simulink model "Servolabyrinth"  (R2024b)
settings: Solver=FixedStepAuto  StartTime=0.0  StopTime=inf  FixedStep=0.01  RelTol=1e-3  EnableMultiTasking=on
libraries: arduinolib x8

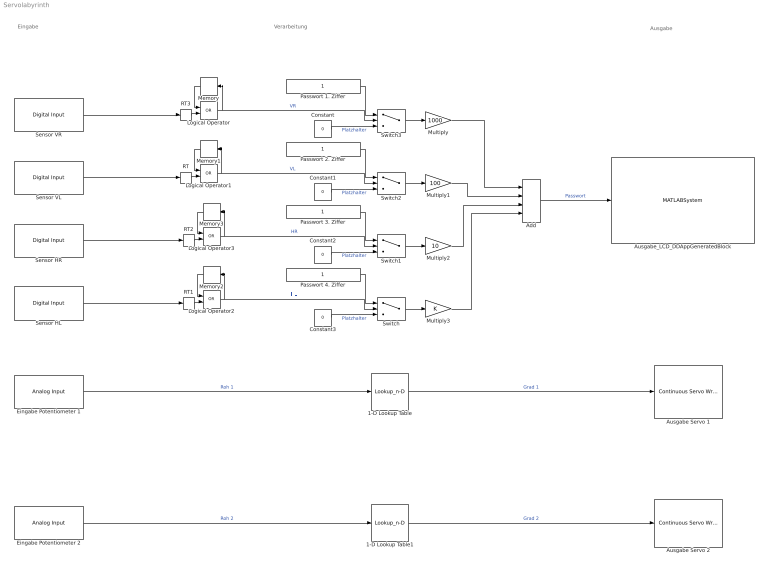
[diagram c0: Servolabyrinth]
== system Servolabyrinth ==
  note: Ausgabe
  note: Verarbeitung
  note: Eingabe
  1-D Lookup Table : Lookup_n-D  NumberOfTableDimensions=1  BreakpointsForDimension1=[0;1023]  Table=[60;110]  InterpMethod=Linear Lagrange  ExtrapMethod=Clip  InternalRulePriority=Speed  RndMeth=Simplest
  1-D Lookup Table1 : Lookup_n-D  NumberOfTableDimensions=1  BreakpointsForDimension1=[0;1023]  Table=[60;110]  InterpMethod=Linear Lagrange  ExtrapMethod=Clip  InternalRulePriority=Speed  RndMeth=Simplest
  Add : Sum  Inputs=++++  OutDataTypeStr=int16
  Ausgabe Servo 1 : arduinolib/Continuous Servo Write  pinNumber=7  ServoIndex=0  blockPlatform=ARDUINO
  Ausgabe Servo 2 : arduinolib/Continuous Servo Write  pinNumber=8  ServoIndex=1  blockPlatform=ARDUINO
  Ausgabe_LCD_DDAppGeneratedBlock : MATLABSystem  System=Ausgabe_LCD  BlockParameter=int16( 0 )  SampleTime=-1
  Constant{,1..3} (4 alike) : Constant  Value=0  OutDataTypeStr=int16
  Eingabe Potentiometer 1 : arduinolib/Analog Input  pinNumber=0  ReadResultsOnly=off  ConversionTriggerSource=Software  ExternalTriggerType=uint32( 0 )  OutputDataType=uint16  EnableConversionCompleteNotify=off  EnableOuputStatus=off  SampleTime=-1  blockPlatform=arduino
  Eingabe Potentiometer 2 : arduinolib/Analog Input  pinNumber=1  ReadResultsOnly=off  ConversionTriggerSource=Software  ExternalTriggerType=uint32( 0 )  OutputDataType=uint16  EnableConversionCompleteNotify=off  EnableOuputStatus=off  SampleTime=-1  blockPlatform=arduino
  Logical Operator{,1..3} (4 alike) : Logic  Operator=OR  AllPortsSameDT=off  OutDataTypeStr=boolean
  Memory{,1..3} (4 alike) : Memory
  Multiply : Gain  Gain=1000  OutDataTypeStr=uint16
  Multiply1 : Gain  Gain=100  OutDataTypeStr=int16
  Multiply2 : Gain  Gain=10  OutDataTypeStr=int16
  Multiply3 : Gain  OutDataTypeStr=int16
  Passwort 1. Ziffer : Constant  OutDataTypeStr=int16
  Passwort 2. Ziffer : Constant  OutDataTypeStr=int16
  Passwort 3. Ziffer : Constant  OutDataTypeStr=int16
  Passwort 4. Ziffer : Constant  OutDataTypeStr=int16
  RT{,1..3} (4 alike) : RateTransition  OutPortSampleTime=0.01
  Sensor HL : arduinolib/Digital Input  pinNumber=13  mode=Default  Direction=input  SampleTime=0.1  blockPlatform=arduino
  Sensor HR : arduinolib/Digital Input  pinNumber=12  mode=Default  Direction=input  SampleTime=0.1  blockPlatform=arduino
  Sensor VL : arduinolib/Digital Input  pinNumber=11  mode=Default  Direction=input  SampleTime=0.1  blockPlatform=arduino
  Sensor VR : arduinolib/Digital Input  pinNumber=10  mode=Default  Direction=input  SampleTime=0.1  blockPlatform=arduino
  Switch{,1..3} (4 alike) : Switch  Criteria=u2 > Threshold
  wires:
  Eingabe Potentiometer 1/1 -> 1-D Lookup Table/1  "Roh 1"
  1-D Lookup Table/1 -> Ausgabe Servo 1/1  "Grad 1"
  1-D Lookup Table1/1 -> Ausgabe Servo 2/1  "Grad 2"
  Eingabe Potentiometer 2/1 -> 1-D Lookup Table1/1  "Roh 2"
  Logical Operator/1 -> Switch3/2, Memory/1  "VR"
  Memory/1 -> Logical Operator/1
  Memory1/1 -> Logical Operator1/1
  Sensor VL/1 -> RT/1
  Logical Operator1/1 -> Switch2/2, Memory1/1  "VL"
  Logical Operator3/1 -> Switch1/2, Memory3/1  "HR"
  Sensor HR/1 -> RT2/1
  Memory3/1 -> Logical Operator3/1
  Memory2/1 -> Logical Operator2/1
  Sensor HL/1 -> RT1/1
  Logical Operator2/1 -> Switch/2, Memory2/1  "HL"
  Sensor VR/1 -> RT3/1
  RT/1 -> Logical Operator1/2
  RT1/1 -> Logical Operator2/2
  RT2/1 -> Logical Operator3/2
  Constant/1 -> Switch3/3  "Platzhalter"
  Constant2/1 -> Switch1/3  "Platzhalter"
  Constant1/1 -> Switch2/3  "Platzhalter"
  Constant3/1 -> Switch/3  "Platzhalter"
  Passwort 1. Ziffer/1 -> Switch3/1
  Passwort 2. Ziffer/1 -> Switch2/1
  Passwort 3. Ziffer/1 -> Switch1/1
  Passwort 4. Ziffer/1 -> Switch/1
  Switch3/1 -> Multiply/1
  Switch2/1 -> Multiply1/1
  Switch1/1 -> Multiply2/1
  Switch/1 -> Multiply3/1
  Multiply/1 -> Add/1
  Multiply1/1 -> Add/2
  Multiply2/1 -> Add/3
  Multiply3/1 -> Add/4
  RT3/1 -> Logical Operator/2
  Add/1 -> Ausgabe_LCD_DDAppGeneratedBlock/1  "Passwort"
